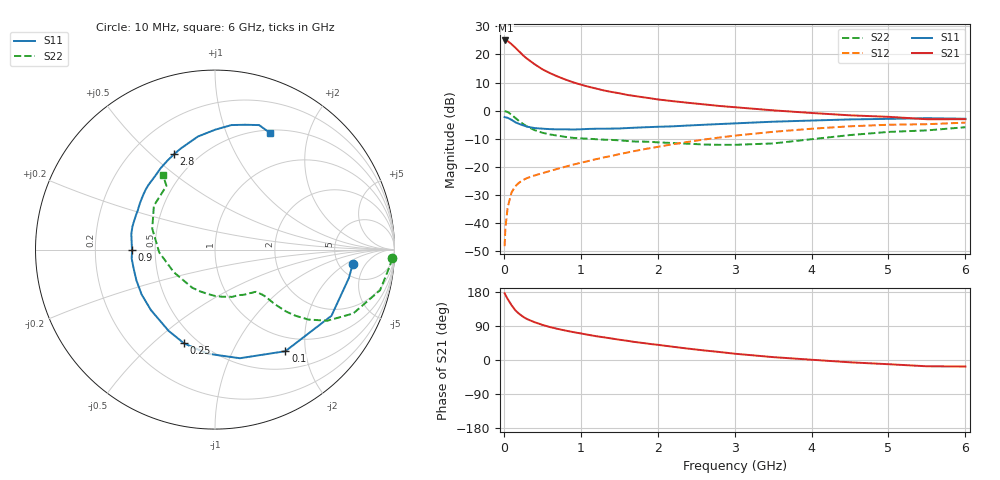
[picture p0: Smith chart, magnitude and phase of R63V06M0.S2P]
! SIEMENS Small Signal Semiconductors
! BFR193
! Si NPN RF Bipolar Junction Transistor in SOT23
! VCE = 3 V  IC = 6 mA
! Common Emitter S-Parameters:  May  1996
# GHz  S  MA  R  50
!  f  S11  S21  S12  S22
! GHz  MAG  ANG  MAG  ANG  MAG  ANG  MAG  ANG
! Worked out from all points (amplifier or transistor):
!   36 points, 10 MHz to 6 GHz, reference 50 ohm
!   highest |S21| = 25.0 dB at 20 MHz (marker M1)
!   |S21| within 3 dB of that: start of sweep to 165.3 MHz
!   unconditionally stable (mu >= 1): 849.7 MHz to 2.027 GHz
!   at 250 MHz: K = 0.48, MSG = 22.2 dB, |S12| = -24.7 dB
!   at 1.4 GHz: K = 1.06, MAG = 9.9 dB, |S12| = -16.1 dB
!   at 6 GHz: K = 0.96, MSG = 0.6 dB, |S12| = -4.2 dB
!   lowest NFmin = 1.20 dB at 450 MHz
!   S11 on the Smith chart (normalised r, x): 10 MHz: 6.64, -2.69; 100 MHz: 0.76, -1.64; 250 MHz: 0.42, -0.63; 900 MHz: 0.37, -0.00; 2.8 GHz: 0.37, +0.59; 6 GHz: 0.53, +1.43
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0.01  0.7716 -6.1  17.69 176.2  0.0039 88.6  0.9892 -2.8
0.02  0.7625 -12.0  17.74 172.0  0.0081 84.7  0.9772 -5.6
0.05  0.7464 -29.6  17.32 160.8  0.0193 75.7  0.9473 -13.8
0.1  0.6886 -55.3  15.24 144.7  0.0351 65.5  0.8485 -24.8
0.15  0.6209 -77.1  13.17 131.0  0.0455 57.6  0.7411 -32.3
0.2  0.5815 -94.0  11.29 121.6  0.0527 53.3  0.6508 -36.8
0.25  0.5501 -108.3  9.641 114.2  0.0585 50.8  0.5806 -39.4
0.3  0.5214 -119.7  8.443 108.1  0.0633 49.8  0.5273 -41.0
0.4  0.4909 -136.7  6.706 99.7  0.0706 49.7  0.4507 -42.4
0.5  0.4792 -148.6  5.459 92.8  0.0773 50.5  0.4059 -42.8
0.6  0.4701 -158.8  4.651 86.9  0.0849 51.8  0.3783 -43.1
0.7  0.4653 -167.0  4.051 82.1  0.0927 53.5  0.3596 -43.8
0.9  0.4624 -179.6  3.201 73.7  0.1097 56.4  0.3285 -45.8
1.1  0.4743 169.4  2.672 66.4  0.1275 58.3  0.3172 -49.3
1.3  0.4781 160.2  2.292 59.9  0.1478 59.0  0.3053 -53.1
1.6  0.491 148.6  1.913 50.8  0.1799 59.4  0.2899 -60.8
2.2  0.5274 129.6  1.477 34.9  0.2539 56.1  0.266 -80.9
2.8  0.5786 113.2  1.215 21.2  0.333 49.5  0.2471 -109.6
3.5  0.6372 98.6  1.015 7.6  0.4211 38.7  0.2617 -151.2
4.5  0.6998 82.5  0.827 -6.1  0.5278 22.6  0.3687 161.5
5.5  0.7359 70.5  0.705 -16.6  0.5754 6.0  0.4465 127.3
6  0.7192 65.0  0.706 -17.2  0.6132 1.1  0.5083 124.8
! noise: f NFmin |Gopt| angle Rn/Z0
0.45  1.2  0.25  114  0.13
0.9  1.25  0.37  150  0.12
1.8  2  0.55  -158  0.12
